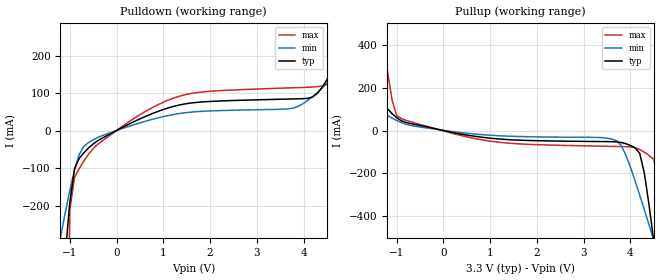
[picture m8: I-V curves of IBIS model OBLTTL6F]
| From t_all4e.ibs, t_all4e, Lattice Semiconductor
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|   OBLTTL6F
[Model]   OBLTTL6F
Model_type   Output
Polarity   Non-Inverting
C_comp   2pF   2pF   2pF
[Temperature Range]   25.0000   125.0000   -40.0000
[Voltage Range]   3.3000V   3.0000V   3.6000V
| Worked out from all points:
|   slope of the pulldown table from 0 to 0.495 V, typ, clamps not added: 16.1 ohm
|   slope of the pullup table from 0 to 0.495 V, typ, clamps not added: 23.4 ohm
[Pulldown]
|voltage   I(typ)   I(min)   I(max)
-3.3V     -4.436A    -1.817A    -40.52A
-1.2V     -495.4mA   -285.6mA   -2.518A
-1.1V     -333.9mA   -220.6mA   -1.039A
-900mV    -102.6mA   -106.1mA   -124.8mA
-800mV    -74.67mA   -64.3mA    -101.9mA
600mV     36.53mA    24.07mA    49.56mA
3.8V      84.32mA    60.53mA    114.1mA
4.6V      158mA      139.6mA    130.7mA
4.8V      207.7mA    168.8mA    333.2mA
5.1V      290.8mA    217.3mA    813.3mA
5.4V      381.5mA    270mA      1.325A
6.6V      773.3mA    501.2mA    3.461A
[Pullup]
|voltage   I(typ)   I(min)   I(max)
-3.3V     752.9mA    436.3mA    3.973A
-2.5V     488.3mA    278.6mA    2.529A
-1.4V     155.1mA    96.47mA    603.1mA
-1V       59.98mA    47.2mA     69.78mA
-800mV    37.72mA    29.55mA    47.83mA
3.6V      -52.17mA   -39.93mA   -74.27mA
4.1V      -80.98mA   -235.7mA   -80.58mA
4.3V      -200.9mA   -372.2mA   -101.3mA
4.5V      -517.8mA   -513.7mA   -135.4mA
4.6V      -693.7mA   -585.4mA   -222mA
4.7V      -873.8mA   -657.6mA   -1.058A
6.6V      -4.462A    -2.062A    -35.02A
[Ramp]
| variable   typ   min   max
dV/dt_r   1.2314/0.3418ns   0.8318/0.5486ns   1.5920/0.1917ns
dV/dt_f   1.4786/0.4245ns   1.1737/0.8814ns   1.7342/0.2230ns
